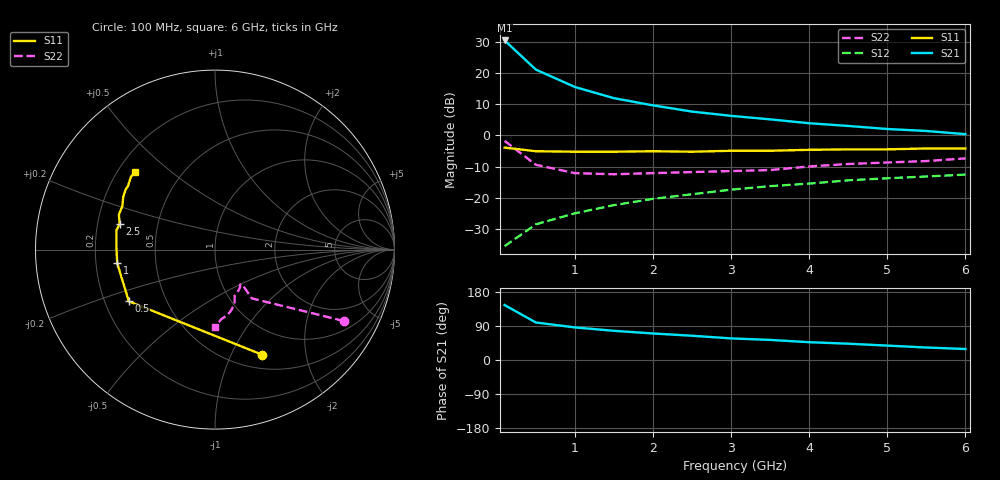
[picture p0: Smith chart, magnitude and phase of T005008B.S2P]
!AT-00500
!S-PARAMETERS at Vce=8V  Ic=20mA.
!OBSOLETED Feb 1994 - nearest replacement: AT-41400
# ghz s ma r 50
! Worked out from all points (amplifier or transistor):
!   13 points, 100 MHz to 6 GHz, reference 50 ohm
!   highest |S21| = 30.4 dB at 100 MHz (marker M1)
!   |S21| within 3 dB of that: start of sweep to 228.8 MHz
!   unconditionally stable (mu >= 1): 1.012 GHz to 5.003 GHz
!   at 1 GHz: K = 1.00, MSG = 20.2 dB, |S12| = -24.9 dB
!   at 3 GHz: K = 1.12, MAG = 9.7 dB, |S12| = -17.3 dB
!   at 6 GHz: K = 0.96, MSG = 6.5 dB, |S12| = -12.5 dB
!   S11 on the Smith chart (normalised r, x): 100 MHz: 0.66, -1.32; 500 MHz: 0.30, -0.25; 1 GHz: 0.29, -0.06; 2.5 GHz: 0.29, +0.12; 6 GHz: 0.27, +0.38
0.1  0.64 -66.0  33.05 145.0  0.017 65.0  0.82 -29.0
0.5  0.56 -149.0  11.31 99.0  0.038 52.0  0.34 -53.0
1  0.55 -172.0  5.96 86.0  0.057 61.0  0.25 -52.0
1.5  0.55 178.0  3.95 77.0  0.077 66.0  0.24 -54.0
2  0.56 169.0  3.03 70.0  0.097 68.0  0.25 -56.0
2.5  0.55 165.0  2.41 64.0  0.115 69.0  0.26 -59.0
3  0.57 160.0  2.06 57.0  0.136 69.0  0.27 -63.0
3.5  0.57 155.0  1.81 53.0  0.155 70.0  0.28 -67.0
4  0.59 150.0  1.57 47.0  0.17 69.0  0.32 -70.0
4.5  0.6 146.0  1.42 43.0  0.192 69.0  0.35 -75.0
5  0.6 144.0  1.27 38.0  0.207 62.0  0.37 -79.0
5.5  0.62 139.0  1.18 33.0  0.221 68.0  0.39 -85.0
6  0.62 136.0  1.05 29.0  0.237 68.0  0.43 -90.0
